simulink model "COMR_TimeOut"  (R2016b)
settings: Solver=FixedStepDiscrete  StartTime=0.0  StopTime=10.0  FixedStep=0.01  RelTol=1e-3  EnableMultiTasking=on
undefined symbols (not defined in the file or in its folder): bin2dec, COMR_cntObcTmtDiag_CW, COMR_cntVcu2A3TmtDiag_CW, COMR_flgTmtCAB_C, COMR_numPackVcuMsg_C, COMR_tiBusoffDiagEna_C, COMR_tiCabMsgTmt_C, COMR_tiCSCMsgTmt_C, COMR_tiGWMsg050Tmt_C, COMR_tiGWMsgTmt_C, COMR_tiHv638MsgTmt_C, COMR_tiMcuMsgTmt_C, COMR_tiObcMsgTmt_C, COMR_tiPackVcuMsgTmt_C, COMR_tiPwrupDiagEna_C, COMR_tiTmtBase_C, COMR_tiVcuMsgTmt_C, COMR_UAESFltDiagDisbl_C
libraries: simulink x167
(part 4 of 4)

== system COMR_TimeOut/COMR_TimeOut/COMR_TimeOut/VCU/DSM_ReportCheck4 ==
  note: Fault report to diagnostic management system
  Dfc_id_nv : Inport  OutDataTypeStr=uint8
  Err : Inport  Port=2
  Heal : Inport  Port=3
  Bit Clear1 : simulink/Logic and Bit Operations/Bit Clear  iBit=4
  Bit Clear2 : simulink/Logic and Bit Operations/Bit Clear  iBit=3
  Bit Set : simulink/Logic and Bit Operations/Bit Set  iBit=4
  Bit Set1 : simulink/Logic and Bit Operations/Bit Set  iBit=3
  Bit Set2 : simulink/Logic and Bit Operations/Bit Set  iBit=3
  Bit Set4 : simulink/Logic and Bit Operations/Bit Set  iBit=7
  Constant1 : Constant  Value=0  OutDataTypeStr=uint8
  Constant7 : Constant  Value=0  OutDataTypeStr=boolean
  Delay2 : Delay  DelayLength=1  InitialCondition=1
  Delay3 : Delay  DelayLength=1  InitialCondition=0
  Logical Operator : Logic  Operator=OR  AllPortsSameDT=off  OutDataTypeStr=boolean
  Switch{1..4} (4 alike) : Switch  Criteria=u2 ~= 0
  Dfc_id : Outport  OutDataTypeStr=uint8
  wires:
  Dfc_id_nv/1 -> Bit Clear2/1, Bit Set4/1, Bit Clear1/1
  Bit Set4/1 -> Bit Set/1
  Constant7/1 -> Delay2/1
  Delay2/1 -> Switch2/2
  Switch3/1 -> Switch2/3
  Bit Clear2/1 -> Switch2/1
  Switch2/1 -> Delay3/1, Switch1/1
  Bit Set1/1 -> Switch3/1
  Bit Set/1 -> Bit Set1/1
  Switch4/1 -> Switch3/3
  Err/1 -> Logical Operator/2, Switch3/2
  Bit Set2/1 -> Switch4/1
  Bit Clear1/1 -> Bit Set2/1
  Delay3/1 -> Switch4/3
  Heal/1 -> Logical Operator/1, Switch4/2
  Logical Operator/1 -> Switch1/2
  Constant1/1 -> Switch1/3
  Switch1/1 -> Dfc_id/1

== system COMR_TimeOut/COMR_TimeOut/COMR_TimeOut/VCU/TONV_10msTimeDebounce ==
  note: Turn On Delay Time Deboune
  u : Inport
  T : Inport  Port=2
  Add : Sum
  Constant1 : Constant  Value=0  OutDataTypeStr=single
  Constant2 : Constant  OutDataTypeStr=uint8
  Constant3 : Constant  Value=0  OutDataTypeStr=uint8
  Constant4 : Constant  Value=0.01  OutDataTypeStr=single
  Delay : Delay  DelayLength=1  InitialCondition=0
  MinMax : MinMax  Inputs=2
  Product : Product  OutMin=[0]  OutMax=[65535]  OutDataTypeStr=single
  Relational Operator : RelationalOperator  Operator=>  OutDataTypeStr=boolean  RndMeth=Simplest
  Switch : Switch  Criteria=u2 ~= 0
  Switch1 : Switch  Criteria=u2 ~= 0
  y : Outport
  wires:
  MinMax/1 -> Add/2
  T/1 -> Relational Operator/2, MinMax/1
  Relational Operator/1 -> y/1
  Delay/1 -> MinMax/2
  Switch/1 -> Add/1
  Product/1 -> Delay/1, Relational Operator/1
  Add/1 -> Product/2
  Constant1/1 -> Switch/3
  Constant4/1 -> Switch/1
  u/1 -> Switch/2, Switch1/2
  Constant2/1 -> Switch1/1
  Constant3/1 -> Switch1/3
  Switch1/1 -> Product/1

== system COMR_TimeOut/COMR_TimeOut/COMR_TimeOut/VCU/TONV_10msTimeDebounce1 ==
  note: Turn On Delay Time Deboune
  u : Inport
  T : Inport  Port=2
  Add : Sum
  Constant1 : Constant  Value=0  OutDataTypeStr=single
  Constant2 : Constant  OutDataTypeStr=uint8
  Constant3 : Constant  Value=0  OutDataTypeStr=uint8
  Constant4 : Constant  Value=0.01  OutDataTypeStr=single
  Delay : Delay  DelayLength=1  InitialCondition=0
  MinMax : MinMax  Inputs=2
  Product : Product  OutMin=[0]  OutMax=[65535]  OutDataTypeStr=single
  Relational Operator : RelationalOperator  Operator=>  OutDataTypeStr=boolean  RndMeth=Simplest
  Switch : Switch  Criteria=u2 ~= 0
  Switch1 : Switch  Criteria=u2 ~= 0
  y : Outport
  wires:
  MinMax/1 -> Add/2
  T/1 -> Relational Operator/2, MinMax/1
  Relational Operator/1 -> y/1
  Delay/1 -> MinMax/2
  Switch/1 -> Add/1
  Product/1 -> Delay/1, Relational Operator/1
  Add/1 -> Product/2
  Constant1/1 -> Switch/3
  Constant4/1 -> Switch/1
  u/1 -> Switch/2, Switch1/2
  Constant2/1 -> Switch1/1
  Constant3/1 -> Switch1/3
  Switch1/1 -> Product/1

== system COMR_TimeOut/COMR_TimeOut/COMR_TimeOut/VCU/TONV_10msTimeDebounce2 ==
  note: Turn On Delay Time Deboune
  u : Inport
  T : Inport  Port=2
  Add : Sum
  Constant1 : Constant  Value=0  OutDataTypeStr=single
  Constant2 : Constant  OutDataTypeStr=uint8
  Constant3 : Constant  Value=0  OutDataTypeStr=uint8
  Constant4 : Constant  Value=0.01  OutDataTypeStr=single
  Delay : Delay  DelayLength=1  InitialCondition=0
  MinMax : MinMax  Inputs=2
  Product : Product  OutMin=[0]  OutMax=[65535]  OutDataTypeStr=single
  Relational Operator : RelationalOperator  Operator=>  OutDataTypeStr=boolean  RndMeth=Simplest
  Switch : Switch  Criteria=u2 ~= 0
  Switch1 : Switch  Criteria=u2 ~= 0
  y : Outport
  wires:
  MinMax/1 -> Add/2
  T/1 -> Relational Operator/2, MinMax/1
  Relational Operator/1 -> y/1
  Delay/1 -> MinMax/2
  Switch/1 -> Add/1
  Product/1 -> Delay/1, Relational Operator/1
  Add/1 -> Product/2
  Constant1/1 -> Switch/3
  Constant4/1 -> Switch/1
  u/1 -> Switch/2, Switch1/2
  Constant2/1 -> Switch1/1
  Constant3/1 -> Switch1/3
  Switch1/1 -> Product/1

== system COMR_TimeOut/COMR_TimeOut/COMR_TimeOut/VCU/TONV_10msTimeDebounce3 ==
  note: Turn On Delay Time Deboune
  u : Inport
  T : Inport  Port=2
  Add : Sum
  Constant1 : Constant  Value=0  OutDataTypeStr=single
  Constant2 : Constant  OutDataTypeStr=uint8
  Constant3 : Constant  Value=0  OutDataTypeStr=uint8
  Constant4 : Constant  Value=0.01  OutDataTypeStr=single
  Delay : Delay  DelayLength=1  InitialCondition=0
  MinMax : MinMax  Inputs=2
  Product : Product  OutMin=[0]  OutMax=[65535]  OutDataTypeStr=single
  Relational Operator : RelationalOperator  Operator=>  OutDataTypeStr=boolean  RndMeth=Simplest
  Switch : Switch  Criteria=u2 ~= 0
  Switch1 : Switch  Criteria=u2 ~= 0
  y : Outport
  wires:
  MinMax/1 -> Add/2
  T/1 -> Relational Operator/2, MinMax/1
  Relational Operator/1 -> y/1
  Delay/1 -> MinMax/2
  Switch/1 -> Add/1
  Product/1 -> Delay/1, Relational Operator/1
  Add/1 -> Product/2
  Constant1/1 -> Switch/3
  Constant4/1 -> Switch/1
  u/1 -> Switch/2, Switch1/2
  Constant2/1 -> Switch1/1
  Constant3/1 -> Switch1/3
  Switch1/1 -> Product/1

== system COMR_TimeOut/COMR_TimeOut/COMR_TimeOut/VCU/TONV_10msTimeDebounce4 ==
  note: Turn On Delay Time Deboune
  u : Inport
  T : Inport  Port=2
  Add : Sum
  Constant1 : Constant  Value=0  OutDataTypeStr=single
  Constant2 : Constant  OutDataTypeStr=uint8
  Constant3 : Constant  Value=0  OutDataTypeStr=uint8
  Constant4 : Constant  Value=0.01  OutDataTypeStr=single
  Delay : Delay  DelayLength=1  InitialCondition=0
  MinMax : MinMax  Inputs=2
  Product : Product  OutMin=[0]  OutMax=[65535]  OutDataTypeStr=single
  Relational Operator : RelationalOperator  Operator=>  OutDataTypeStr=boolean  RndMeth=Simplest
  Switch : Switch  Criteria=u2 ~= 0
  Switch1 : Switch  Criteria=u2 ~= 0
  y : Outport
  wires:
  Switch1/1 -> Product/1
  Constant3/1 -> Switch1/3
  Constant2/1 -> Switch1/1
  u/1 -> Switch1/2, Switch/2
  Constant4/1 -> Switch/1
  Constant1/1 -> Switch/3
  Add/1 -> Product/2
  Product/1 -> Relational Operator/1, Delay/1
  Switch/1 -> Add/1
  Delay/1 -> MinMax/2
  Relational Operator/1 -> y/1
  T/1 -> MinMax/1, Relational Operator/2
  MinMax/1 -> Add/2

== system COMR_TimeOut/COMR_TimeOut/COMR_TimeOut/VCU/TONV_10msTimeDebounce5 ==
  note: Turn On Delay Time Deboune
  u : Inport
  T : Inport  Port=2
  Add : Sum
  Constant1 : Constant  Value=0  OutDataTypeStr=single
  Constant2 : Constant  OutDataTypeStr=uint8
  Constant3 : Constant  Value=0  OutDataTypeStr=uint8
  Constant4 : Constant  Value=0.01  OutDataTypeStr=single
  Delay : Delay  DelayLength=1  InitialCondition=0
  MinMax : MinMax  Inputs=2
  Product : Product  OutMin=[0]  OutMax=[65535]  OutDataTypeStr=single
  Relational Operator : RelationalOperator  Operator=>  OutDataTypeStr=boolean  RndMeth=Simplest
  Switch : Switch  Criteria=u2 ~= 0
  Switch1 : Switch  Criteria=u2 ~= 0
  y : Outport
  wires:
  MinMax/1 -> Add/2
  T/1 -> Relational Operator/2, MinMax/1
  Relational Operator/1 -> y/1
  Delay/1 -> MinMax/2
  Switch/1 -> Add/1
  Product/1 -> Delay/1, Relational Operator/1
  Add/1 -> Product/2
  Constant1/1 -> Switch/3
  Constant4/1 -> Switch/1
  u/1 -> Switch/2, Switch1/2
  Constant2/1 -> Switch1/1
  Constant3/1 -> Switch1/3
  Switch1/1 -> Product/1

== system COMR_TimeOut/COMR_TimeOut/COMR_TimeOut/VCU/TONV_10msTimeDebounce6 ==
  note: Turn On Delay Time Deboune
  u : Inport
  T : Inport  Port=2
  Add : Sum
  Constant1 : Constant  Value=0  OutDataTypeStr=single
  Constant2 : Constant  OutDataTypeStr=uint8
  Constant3 : Constant  Value=0  OutDataTypeStr=uint8
  Constant4 : Constant  Value=0.01  OutDataTypeStr=single
  Delay : Delay  DelayLength=1  InitialCondition=0
  MinMax : MinMax  Inputs=2
  Product : Product  OutMin=[0]  OutMax=[65535]  OutDataTypeStr=single
  Relational Operator : RelationalOperator  Operator=>  OutDataTypeStr=boolean  RndMeth=Simplest
  Switch : Switch  Criteria=u2 ~= 0
  Switch1 : Switch  Criteria=u2 ~= 0
  y : Outport
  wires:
  MinMax/1 -> Add/2
  T/1 -> Relational Operator/2, MinMax/1
  Relational Operator/1 -> y/1
  Delay/1 -> MinMax/2
  Switch/1 -> Add/1
  Product/1 -> Delay/1, Relational Operator/1
  Add/1 -> Product/2
  Constant1/1 -> Switch/3
  Constant4/1 -> Switch/1
  u/1 -> Switch/2, Switch1/2
  Constant2/1 -> Switch1/1
  Constant3/1 -> Switch1/3
  Switch1/1 -> Product/1

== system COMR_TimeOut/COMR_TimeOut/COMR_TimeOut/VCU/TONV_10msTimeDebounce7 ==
  note: Turn On Delay Time Deboune
  u : Inport
  T : Inport  Port=2
  Add : Sum
  Constant1 : Constant  Value=0  OutDataTypeStr=single
  Constant2 : Constant  OutDataTypeStr=uint8
  Constant3 : Constant  Value=0  OutDataTypeStr=uint8
  Constant4 : Constant  Value=0.01  OutDataTypeStr=single
  Delay : Delay  DelayLength=1  InitialCondition=0
  MinMax : MinMax  Inputs=2
  Product : Product  OutMin=[0]  OutMax=[65535]  OutDataTypeStr=single
  Relational Operator : RelationalOperator  Operator=>  OutDataTypeStr=boolean  RndMeth=Simplest
  Switch : Switch  Criteria=u2 ~= 0
  Switch1 : Switch  Criteria=u2 ~= 0
  y : Outport
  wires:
  Switch1/1 -> Product/1
  Constant3/1 -> Switch1/3
  Constant2/1 -> Switch1/1
  u/1 -> Switch1/2, Switch/2
  Constant4/1 -> Switch/1
  Constant1/1 -> Switch/3
  Add/1 -> Product/2
  Product/1 -> Relational Operator/1, Delay/1
  Switch/1 -> Add/1
  Delay/1 -> MinMax/2
  Relational Operator/1 -> y/1
  T/1 -> MinMax/1, Relational Operator/2
  MinMax/1 -> Add/2

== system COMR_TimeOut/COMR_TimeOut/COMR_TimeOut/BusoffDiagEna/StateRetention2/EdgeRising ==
  u : Inport
  Delay1 : Delay  DelayLength=1  InitialCondition=1
  Logical Operator3 : Logic  Operator=NOT  AllPortsSameDT=off  OutDataTypeStr=boolean
  Logical Operator4 : Logic  AllPortsSameDT=off  OutDataTypeStr=boolean
  y : Outport
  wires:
  Delay1/1 -> Logical Operator3/1
  u/1 -> Logical Operator4/2, Delay1/1
  Logical Operator3/1 -> Logical Operator4/1
  Logical Operator4/1 -> y/1

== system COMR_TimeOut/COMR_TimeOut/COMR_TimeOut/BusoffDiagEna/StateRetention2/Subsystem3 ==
  set : Inport
  clear : Inport  Port=2
  Delay : Delay  DelayLength=1  InitialCondition=0
  Logical Operator : Logic  Operator=OR  AllPortsSameDT=off  OutDataTypeStr=boolean
  Logical Operator1 : Logic  Operator=NOT  AllPortsSameDT=off  OutDataTypeStr=boolean
  Logical Operator4 : Logic  AllPortsSameDT=off  OutDataTypeStr=boolean
  Logical Operator5 : Logic  Operator=NOT  AllPortsSameDT=off  OutDataTypeStr=boolean
  Q : Outport
  _Q : Outport  Port=2
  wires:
  Delay/1 -> Logical Operator/1
  Logical Operator4/1 -> Q/1, Delay/1, Logical Operator1/1
  Logical Operator/1 -> Logical Operator4/1
  Logical Operator5/1 -> Logical Operator4/2
  clear/1 -> Logical Operator5/1
  set/1 -> Logical Operator/2
  Logical Operator1/1 -> _Q/1

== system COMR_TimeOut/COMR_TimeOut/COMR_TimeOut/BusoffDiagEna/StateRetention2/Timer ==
  En : Inport
  Ts : Inport  Port=2
  Rst : Inport  Port=3
  Vst : Inport  Port=4
  Add : Sum
  Constant5 : Constant  Value=single(0)  OutDataTypeStr=single
  Switch1 : Switch  Criteria=u2 ~= 0
  Switch2 : Switch  Criteria=u2 ~= 0
  Unit Delay : UnitDelay  SampleTime=-1
  Timer : Outport
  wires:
  Unit Delay/1 -> Add/2
  Rst/1 -> Switch1/2
  En/1 -> Switch2/2
  Ts/1 -> Switch2/1
  Constant5/1 -> Switch2/3
  Switch2/1 -> Add/1
  Vst/1 -> Switch1/1
  Switch1/1 -> Timer/1, Unit Delay/1
  Add/1 -> Switch1/3

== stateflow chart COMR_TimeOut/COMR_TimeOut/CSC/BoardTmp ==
  state CSC_Timeout
    (default) -> (junction 3)
    (junction 3) -> (junction 18) : [BSWBoardTempMsgRx[0] == true... || BSWBoardTempMsgRx[1] == true]
    (junction 18) -> (junction 20) : {COMR_flgTmtBoardTmp = false;}
    (junction 3) -> (junction 32) : [ (BSWBoardTempMsgRx[0]) == false... &&(BSWBoardTempMsgRx[1]) == false]
    (junction 32) -> (junction 8) : {COMR_flgTmtBoardTmp = true;}
    (junction 20) -> (junction 8)
    (junction 8) -> (junction 11)
  (default) -> CSC_Timeout
  CSC_Timeout -> CSC_Timeout
  data: BSWBoardTempMsgRx input; COMR_flgTmtBoardTmp output; i local uint8

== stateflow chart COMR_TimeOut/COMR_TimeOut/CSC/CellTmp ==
  state CSC_Timeout
    (default) -> (junction 3)
    (junction 3) -> (junction 18) : [((BSWCellTempMsgRx[0] == true)...  || (BSWCellTempMsgRx[1] == true)...  || (BSWCellTempMsgRx[2] == true))...  && ((BSWCellTempMsgRx[3] == true)...  || (BSWCellTempMsgRx[4] == true)...  || (BSWCellTempMsgRx[5] == true))]
    (junction 18) -> (junction 20) : {COMR_flgTmtCellTmp = false;}
    (junction 3) -> (junction 32) : [ ((BSWCellTempMsgRx[0] == false)...  && (BSWCellTempMsgRx[1] == false)...  && (BSWCellTempMsgRx[2] == false))... || ((BSWCellTempMsgRx[3] == false)...  && (BSWCellTempMsgRx[4] == false)...  && (BSWCellTempMsgRx[5] == false))]
    (junction 32) -> (junction 8) : {COMR_flgTmtCellTmp = true;}
    (junction 20) -> (junction 8)
    (junction 8) -> (junction 38)
  (default) -> CSC_Timeout
  CSC_Timeout -> CSC_Timeout
  data: BSWCellTempMsgRx input; COMR_flgTmtCellTmp output; i local uint8

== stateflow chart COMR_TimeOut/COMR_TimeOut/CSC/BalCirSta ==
  state CSC_Timeout
    (default) -> (junction 3)
    (junction 3) -> (junction 18) : [BSWCellBalanceCircuitStatusMsgRx[0] == true... ||BSWCellBalanceCircuitStatusMsgRx[1] == true]
    (junction 18) -> (junction 20) : {COMR_flgTmtBalCirSta = false;}
    (junction 3) -> (junction 34) : [ (BSWCellBalanceCircuitStatusMsgRx[0]) == false... && (BSWCellBalanceCircuitStatusMsgRx[1]) == false]
    (junction 34) -> (junction 8) : {COMR_flgTmtBalCirSta = true;}
    (junction 20) -> (junction 8)
    (junction 8) -> (junction 11)
  (default) -> CSC_Timeout
  CSC_Timeout -> CSC_Timeout
  data: BSWCellBalanceCircuitStatusMsgRx input; COMR_flgTmtBalCirSta output; i local uint8

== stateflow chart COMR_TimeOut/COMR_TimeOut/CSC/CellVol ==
  state CSC_Timeout
    (default) -> (junction 3)
    (junction 3) -> (junction 18)
    (junction 18) -> (junction 20) : [((BSWCellVoltageMsgRx[0] == true)...  || (BSWCellVoltageMsgRx[1] == true)...  || (BSWCellVoltageMsgRx[2] == true)... || (BSWCellVoltageMsgRx[3] == true)... || (BSWCellVoltageMsgRx[4] == true)... || (BSWCellVoltageMsgRx[5] == true)... || (BSWCellVoltageMsgRx[6] == true)... || (BSWCellVoltageMsgRx[7] == true)... || (BSWCellVoltageMsgRx[8] == true)... || (BSWCellVoltageMsgRx[9] == true)... || (BSWCellVoltageMsgRx[10] == true)... || (BSWCellVoltageMsgRx[11] == true))... && ((BSWCellVoltageMsgRx[12] == true)... || (BSWCellVoltageMsgRx[13] == true)... || (BSWCellVoltageMsgRx[14] == true)... || (BSWCellVoltageMsgRx[15] == true)... || (BSWCellVoltageMsgRx[16] == true)... || (BSWCellVoltageMsgRx[17] == true)... || (BSWCellVoltageMsgRx[18] == true)... || (BSWCellVoltageMsgRx[19] == true)... || (BSWCellVoltageMsgRx[20] == true)... || (BSWCellVoltageMsgRx[21] == true)... || (BSWCellVoltageMsgRx[22] == true)... || (BSWCellVoltageMsgRx[23] == true))... ]
    (junction 3) -> (junction 32) : [ ((BSWCellVoltageMsgRx[0] == false) ... && (BSWCellVoltageMsgRx[1] == false) ... && (BSWCellVoltageMsgRx[2] == false)... && (BSWCellVoltageMsgRx[3] == false)... && (BSWCellVoltageMsgRx[4] == false)... && (BSWCellVoltageMsgRx[5] == false)... && (BSWCellVoltageMsgRx[6] == false)... && (BSWCellVoltageMsgRx[7] == false)... && (BSWCellVoltageMsgRx[8] == false)... && (BSWCellVoltageMsgRx[9] == false)... && (BSWCellVoltageMsgRx[10] == false)... && (BSWCellVoltageMsgRx[11] == false))... || ((BSWCellVoltageMsgRx[12] == false)... && (BSWCellVoltageMsgRx[13] == false)... && (BSWCellVoltageMsgRx[14] == false)... && (BSWCellVoltageMsgRx[15] == false)... && (BSWCellVoltageMsgRx[16] == false)... && (BSWCellVoltageMsgRx[17] == false)... && (BSWCellVoltageMsgRx[18] == false)... && (BSWCellVoltageMsgRx[19] == false)... && (BSWCellVoltageMsgRx[20] == false)... && (BSWCellVoltageMsgRx[21] == false)... && (BSWCellVoltageMsgRx[22] == false)... && (BSWCellVoltageMsgRx[23] == false))]
    (junction 32) -> (junction 8) : {COMR_flgTmtCellVol = true;}
    (junction 20) -> (junction 8) : {COMR_flgTmtCellVol = false;}
    (junction 8) -> (junction 37)
  (default) -> CSC_Timeout
  CSC_Timeout -> CSC_Timeout
  data: BSWCellVoltageMsgRx input; COMR_flgTmtCellVol output; i local uint8

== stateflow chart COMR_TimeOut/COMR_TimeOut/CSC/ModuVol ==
  state CSC_Timeout
    (default) -> (junction 3)
    (junction 3) -> (junction 18) : [BSWModuleVoltageMsgRx[0] == true... || BSWModuleVoltageMsgRx[1] == true]
    (junction 18) -> (junction 20) : {COMR_flgTmtModuVol = false;}
    (junction 3) -> (junction 32) : [ (BSWModuleVoltageMsgRx[0] == false)... && (BSWModuleVoltageMsgRx[1] == false)]
    (junction 32) -> (junction 8) : {COMR_flgTmtModuVol = true;}
    (junction 20) -> (junction 8)
    (junction 8) -> (junction 37)
  (default) -> CSC_Timeout
  CSC_Timeout -> CSC_Timeout
  data: BSWModuleVoltageMsgRx input; COMR_flgTmtModuVol output; i local uint8
